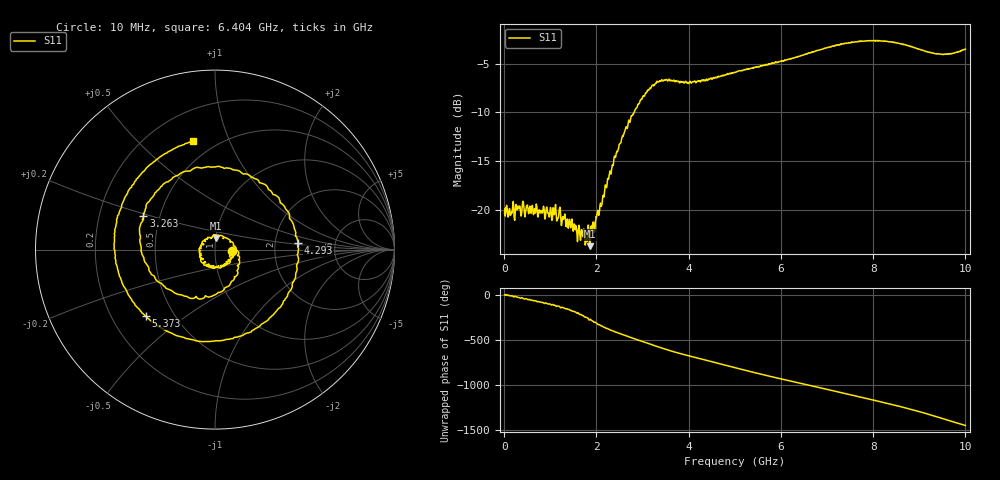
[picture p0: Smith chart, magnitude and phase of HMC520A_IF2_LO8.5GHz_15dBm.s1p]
! Analog Devices, Inc.
! 1 Analog Way
! Wilmington, MA 01887
! http://www.analog.com
! Date:  2021-09-07 NN
! Board Name:  EV1HMC520ALC4 Revision A with HMC520ALC4 installed
! File Description:  S-Parameters for evaluation board without connectors or board loss de-embedded
! File Generation:  Calibrated Network Analyzer
! Chip Part Number:  HMC520A
! Chip Description:  GaAs, MMIC, IQ Mixer
! Chip Frequency:  6 to 10 GHz
! Chip Package:  LCC, 3.9 x 3.9 x 0.9 mm
! Chip State:
!  Temperature:  25C
!  LO Frequency:  8.5GHz
!  LO Power:  15dBm
! Note:
!  Analog Devices supplies this data as a sample of measured data at the evaluation board
!  ports for this product.  Your particular data for this product may vary.
!  Analog Devices reserves the right to change this data at anytime.
!  All lines below in this file are as is from the Network Analyzer.
!Keysight Technologies,N5245A,MY49151104,A.10.65.16
!Date: Wednesday, August 04, 2021 10:53:27
!Correction: S22(Full 2 Port(1,2))
!S1P File: Measurement: S22:
# Hz S  dB  R 50
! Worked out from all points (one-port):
!   1601 points, 10 MHz to 10 GHz, reference 50 ohm
!   lowest |S11| = -23.8 dB at 1.858 GHz (marker M1), VSWR 1.14, Z = 50.1 + j6.51 ohm
!   |S11| at or under -10 dB: start of sweep to 2.818 GHz
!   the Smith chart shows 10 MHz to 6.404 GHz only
!   S11 on the Smith chart (normalised r, x): 10 MHz: 1.21, -0.02; 3.263 GHz: 0.40, +0.19; 4.293 GHz: 2.70, +0.26; 5.373 GHz: 0.35, -0.36; 6.404 GHz: 0.38, +0.74
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1e7  -20.34 -4.3
1.25875e9  -21.12 -141.2
1.85815e9  -23.75 85.0
2.232775e9  -17.34 -14.4
2.5075e9  -13.23 -72.7
2.863394e9  -9.57 -135.8
3.262994e9  -7.12 154.9
3.518988e9  -6.59 111.9
3.75625e9  -6.81 76.7
4.293212e9  -6.68 4.6
4.624131e9  -6.34 -38.4
5.005e9  -5.88 -88.7
5.373381e9  -5.44 -135.9
5.8042e9  -4.92 171.2
6.25375e9  -4.41 118.7
6.4036e9  -4.21 101.5
6.722031e9  -3.76 64.4
7.059194e9  -3.27 24.7
7.277725e9  -3.03 -0.9
7.5025e9  -2.83 -27.4
7.833419e9  -2.65 -66.3
8.114388e9  -2.63 -99.5
8.464038e9  -2.81 -142.2
8.75125e9  -3.12 -179.2
9.1009e9  -3.65 131.6
9.375625e9  -3.97 89.8
9.719031e9  -3.93 35.7
1e10  -3.49 -6.7
